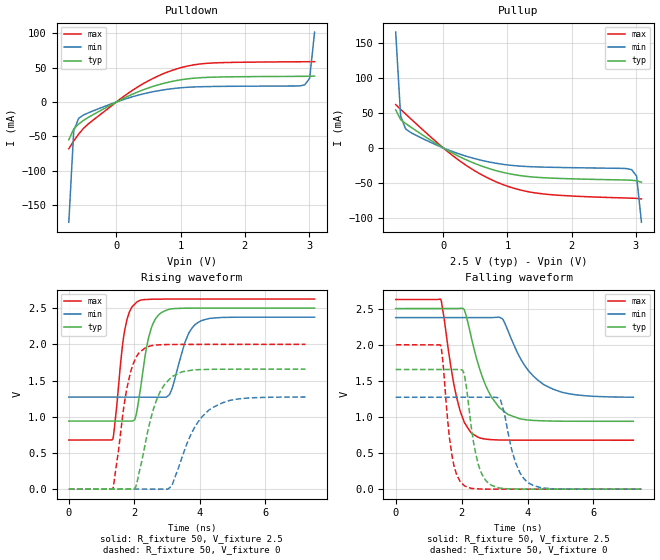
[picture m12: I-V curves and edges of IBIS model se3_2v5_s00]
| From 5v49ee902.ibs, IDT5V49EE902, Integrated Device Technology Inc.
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[Model]   se3_2v5_s00
Model_type   Output
Polarity   Non-Inverting
|   typ   min   max
C_comp   2pF   1.5pF   2.5pF
Vmeas = 1.25V
Rref = 50
Cref = 0
Vref = 1.25V
|   typ   min   max
[Voltage range]   2.5V   2.375V   2.625V
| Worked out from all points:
|   slope of the pulldown table from 0 to 0.375 V, typ, clamps not added: 23.2 ohm
|   slope of the pullup table from 0 to 0.375 V, typ, clamps not added: 21 ohm
|   rising waveform, R_fixture 50, V_fixture 2.5: 20-80 % time 352ps typ, 443ps min, 279ps max; typ from 0.939 V to 2.5 V
|   falling waveform, R_fixture 50, V_fixture 2.5: 20-80 % time 692ps typ, 919ps min, 460ps max; typ from 2.5 V to 0.939 V
|   rising waveform, R_fixture 50, V_fixture 0: 20-80 % time 568ps typ, 793ps min, 399ps max; typ from 0 V to 1.66 V
|   falling waveform, R_fixture 50, V_fixture 0: 20-80 % time 344ps typ, 431ps min, 274ps max; typ from 1.66 V to 0 V
[Pulldown]
|Voltage   I (typ)   I (min)   I (max)
|Note, modeling breaks down at 250mA and above.  This is well beyond the functional   |
|operating range of the device.  Should this scenario occur, catastrophic failure and   |
|possible damage to the device and/or board is of higher concern than the I-V curve   |
|behavior.  The IBIS checker will flag currents in excess of 10A with warnings.  Lines   |
|with currents in excess of 0.35 A have been commented out.  The points still remain|
|available to the user if the user desires to use them.   |
|-2.50000e+00   -4.54709e+01   -3.63694e+01   -6.07959e+01
|-2.42347e+00   -4.32502e+01   -3.46594e+01   -5.77053e+01
|-2.34694e+00   -4.10314e+01   -3.29511e+01   -5.46170e+01
|-2.27041e+00   -3.88148e+01   -3.12446e+01   -5.15313e+01
|-2.19388e+00   -3.66007e+01   -2.95401e+01   -4.84486e+01
|-2.11735e+00   -3.43893e+01   -2.78380e+01   -4.53691e+01
|-2.04082e+00   -3.21809e+01   -2.61384e+01   -4.22934e+01
|-1.96429e+00   -2.99761e+01   -2.44418e+01   -3.92219e+01
|-1.88776e+00   -2.77753e+01   -2.27484e+01   -3.61555e+01
|-1.81122e+00   -2.55791e+01   -2.10589e+01   -3.30948e+01
|-1.73469e+00   -2.33884e+01   -1.93737e+01   -3.00411e+01
|-1.65816e+00   -2.12042e+01   -1.76937e+01   -2.69958e+01
|-1.58163e+00   -1.90279e+01   -1.60198e+01   -2.39607e+01
|-1.50510e+00   -1.68611e+01   -1.43533e+01   -2.09385e+01
|-1.42857e+00   -1.47065e+01   -1.26960e+01   -1.79331e+01
|-1.35204e+00   -1.25675e+01   -1.10500e+01   -1.49501e+01
|-1.27551e+00   -1.04495e+01   -9.41889e+00   -1.19989e+01
|-1.19898e+00   -8.36102e+00   -7.80755e+00   -9.09553e+00
|-1.12245e+00   -6.31683e+00   -6.22400e+00   -6.27207e+00
|-1.04592e+00   -4.34540e+00   -4.68188e+00   -3.60463e+00
|-9.69388e-01   -2.51112e+00   -3.20700e+00   -1.33260e+00
|-8.92857e-01   -9.89892e-01   -1.85502e+00   -2.01598e-01
|-8.16327e-01   -1.92135e-01   -7.61074e-01   -8.24374e-02
-739.8mV  -54.82mA   -174.4mA   -67.73mA
-663.3mV  -39mA      -41.68mA   -56.5mA
-586.7mV  -31.96mA   -23.62mA   -46.47mA
-433.7mV  -22.15mA   -15.6mA    -31.55mA
255.1mV   11.54mA    7.746mA    17.23mA
637.8mV   24.55mA    16.14mA    37.26mA
943.9mV   31.29mA    20.16mA    48.22mA
1.173V    34.28mA    21.72mA    53.44mA
1.48V     36mA       22.52mA    56.56mA
2.934V    37.31mA    24.91mA    58.47mA
3.01V     37.39mA    34.58mA    58.51mA
3.087V    37.69mA    101.5mA    58.57mA
| 3.16327e+00   3.94370e-02   3.90706e-01   5.87161e-02
| 3.23980e+00   5.34568e-02   9.26296e-01   5.92247e-02
| 3.31633e+00   1.87774e-01   1.58657e+00   6.05142e-02
| 3.39286e+00   7.03870e-01   2.30639e+00   6.31621e-02
| 3.46939e+00   1.49288e+00   3.05886e+00   8.17834e-02
| 3.54592e+00   2.39288e+00   3.83148e+00   3.62561e-01
| 3.62245e+00   3.34491e+00   4.61762e+00   1.23059e+00
| 3.69898e+00   4.32602e+00   5.41341e+00   2.35266e+00
| 3.77551e+00   5.32544e+00   6.21640e+00   3.56507e+00
| 3.85204e+00   6.33737e+00   7.02496e+00   4.82041e+00
| 3.92857e+00   7.35834e+00   7.83797e+00   6.10033e+00
| 4.00510e+00   8.38614e+00   8.65458e+00   7.39607e+00
| 4.08163e+00   9.41929e+00   9.47419e+00   8.70278e+00
| 4.15816e+00   1.04567e+01   1.02963e+01   1.00176e+01
| 4.23469e+00   1.14977e+01   1.11206e+01   1.13385e+01
| 4.31122e+00   1.25415e+01   1.19467e+01   1.26642e+01
| 4.38776e+00   1.35879e+01   1.27745e+01   1.39940e+01
| 4.46429e+00   1.46363e+01   1.36036e+01   1.53269e+01
| 4.54082e+00   1.56867e+01   1.44341e+01   1.66626e+01
| 4.61735e+00   1.67386e+01   1.52656e+01   1.80006e+01
| 4.69388e+00   1.77920e+01   1.60982e+01   1.93406e+01
| 4.77041e+00   1.88466e+01   1.69317e+01   2.06823e+01
| 4.84694e+00   1.99024e+01   1.77660e+01   2.20256e+01
| 4.92347e+00   2.09592e+01   1.86011e+01   2.33703e+01
| 5.00000e+00   2.20169e+01   1.94369e+01   2.47161e+01
[Pullup]
|Voltage   I (typ)   I (min)   I (max)
|Note, modeling breaks down at 250mA and above.  This is well beyond the functional   |
|operating range of the device.  Should this scenario occur, catastrophic failure and   |
|possible damage to the device and/or board is of higher concern than the I-V curve   |
|behavior.  The IBIS checker will flag currents in excess of 10A with warnings.  Lines   |
|with currents in excess of 0.35 A have been commented out.  The points still remain|
|available to the user if the user desires to use them.   |
|-2.50000e+00   2.19749e+01   1.80462e+01   2.68494e+01
|-2.42347e+00   2.09176e+01   1.72118e+01   2.55026e+01
|-2.34694e+00   1.98612e+01   1.63782e+01   2.41568e+01
|-2.27041e+00   1.88058e+01   1.55455e+01   2.28121e+01
|-2.19388e+00   1.77516e+01   1.47137e+01   2.14686e+01
|-2.11735e+00   1.66986e+01   1.38831e+01   2.01266e+01
|-2.04082e+00   1.56470e+01   1.30536e+01   1.87861e+01
|-1.96429e+00   1.45970e+01   1.22255e+01   1.74474e+01
|-1.88776e+00   1.35488e+01   1.13989e+01   1.61108e+01
|-1.81122e+00   1.25028e+01   1.05741e+01   1.47767e+01
|-1.73469e+00   1.14592e+01   9.75133e+00   1.34454e+01
|-1.65816e+00   1.04186e+01   8.93094e+00   1.21176e+01
|-1.58163e+00   9.38151e+00   8.11336e+00   1.07941e+01
|-1.50510e+00   8.34872e+00   7.29916e+00   9.47586e+00
|-1.42857e+00   7.32129e+00   6.48907e+00   8.16447e+00
|-1.35204e+00   6.30078e+00   5.68413e+00   6.86214e+00
|-1.27551e+00   5.28938e+00   4.88577e+00   5.57245e+00
|-1.19898e+00   4.29063e+00   4.09609e+00   4.30150e+00
|-1.12245e+00   3.31046e+00   3.31840e+00   3.06092e+00
|-1.04592e+00   2.35988e+00   2.55815e+00   1.87698e+00
|-9.69388e-01   1.46255e+00   1.82528e+00   8.26188e-01
|-8.92857e-01   6.79691e-01   1.14020e+00   1.77018e-01
|-8.16327e-01   1.78301e-01   5.50929e-01   7.20286e-02
-739.8mV  54.64mA    166.3mA    62.19mA
-663.3mV  40.61mA    45.96mA    55.4mA
-586.7mV  35.13mA    27.42mA    48.78mA
-204.1mV  11.53mA    8.292mA    16.47mA
255.1mV   -12.67mA   -8.857mA   -18.54mA
561.2mV   -24.84mA   -17.08mA   -36.7mA
943.9mV   -35.45mA   -23.78mA   -53.18mA
1.25V     -40.42mA   -26.48mA   -61.53mA
1.556V    -42.81mA   -27.59mA   -66.09mA
2.934V    -46.44mA   -31.28mA   -72.19mA
3.01V     -47.21mA   -40.39mA   -72.48mA
3.087V    -49.28mA   -106.7mA   -73.28mA
| 3.16327e+00   -5.35776e-02   -4.94236e-01   -7.58575e-02
| 3.23980e+00   -6.85824e-02   -1.43626e+00   -8.09810e-02
| 3.31633e+00   -2.12479e-01   -2.71822e+00   -8.81300e-02
| 3.39286e+00   -1.02359e+00   -4.15794e+00   -9.69441e-02
| 3.46939e+00   -2.55073e+00   -5.67974e+00   -1.18777e-01
| 3.54592e+00   -4.38708e+00   -7.25021e+00   -4.69271e-01
| 3.62245e+00   -6.35927e+00   -8.85247e+00   -2.14689e+00
| 3.69898e+00   -8.40369e+00   -1.04769e+01   -4.62063e+00
| 3.77551e+00   -1.04921e+01   -1.21177e+01   -7.36117e+00
| 3.85204e+00   -1.26099e+01   -1.37710e+01   -1.02197e+01
| 3.92857e+00   -1.47486e+01   -1.54342e+01   -1.31429e+01
| 4.00510e+00   -1.69029e+01   -1.71053e+01   -1.61066e+01
| 4.08163e+00   -1.90692e+01   -1.87829e+01   -1.90980e+01
| 4.15816e+00   -2.12452e+01   -2.04660e+01   -2.21093e+01
| 4.23469e+00   -2.34289e+01   -2.21537e+01   -2.51357e+01
| 4.31122e+00   -2.56192e+01   -2.38455e+01   -2.81738e+01
| 4.38776e+00   -2.78148e+01   -2.55407e+01   -3.12215e+01
| 4.46429e+00   -3.00151e+01   -2.72389e+01   -3.42769e+01
| 4.54082e+00   -3.22195e+01   -2.89399e+01   -3.73388e+01
| 4.61735e+00   -3.44273e+01   -3.06432e+01   -4.04061e+01
| 4.69388e+00   -3.66382e+01   -3.23486e+01   -4.34782e+01
| 4.77041e+00   -3.88519e+01   -3.40560e+01   -4.65543e+01
| 4.84694e+00   -4.10679e+01   -3.57652e+01   -4.96340e+01
| 4.92347e+00   -4.32862e+01   -3.74759e+01   -5.27168e+01
| 5.00000e+00   -4.55064e+01   -3.91880e+01   -5.58024e+01
[Ramp]
|   typ   min   max
dV/dt_r   0.936/0.352n   0.663/0.443n   1.168/0.279n
dV/dt_f   0.939/0.692n   0.665/0.919n   1.172/0.46n
R_load =   50
[Rising Waveform]
R_fixture = 50
V_fixture = 2.5   |Vcc_typ
V_fixture_min = 2.375 |Vcc_min
V_fixture_max = 2.625 |Vcc_max
C_fixture = 0.0p
| Time   typ   min   max
0s        939.3mV    1.271V     677.7mV
1.339ns   939.3mV    1.271V     689.1mV
1.7ns     939.3mV    1.271V     2.184V
2.089ns   1.104V     1.271V     2.589V
2.429ns   2.082V     1.271V     2.621V
2.816ns   2.435V     1.27V      2.625V
3.073ns   2.485V     1.306V     2.625V
3.534ns   2.499V     2.017V     2.625V
3.97ns    2.5V       2.309V     2.625V
7.5ns     2.5V       2.375V     2.625V
[Falling Waveform]
R_fixture = 50
V_fixture = 2.5   |Vcc_typ
V_fixture_min = 2.375 |Vcc_min
V_fixture_max = 2.625 |Vcc_max
C_fixture = 0.0p
| Time   typ   min   max
0s        2.5V       2.375V     2.625V
1.37ns    2.5V       2.375V     2.627V
1.951ns   2.502V     2.375V     1.087V
2.082ns   2.484V     2.375V     924.2mV
2.457ns   1.802V     2.375V     729.3mV
2.902ns   1.279V     2.375V     685.4mV
3.411ns   1.033V     2.19V      678.8mV
3.913ns   963.2mV    1.713V     678mV
4.495ns   945.1mV    1.446V     677.9mV
7.213ns   939.5mV    1.273V     677.8mV
[Rising Waveform]
R_fixture = 50
V_fixture = 0
C_fixture = 0.0p
| Time   typ   min   max
0s        1.586nV    7.942nV    136.5pV
1.35ns    -13.68nV   8.225nV    10.74mV
1.87ns    -174.4uV   30.88nV    1.592V
2.044ns   31.78mV    -4.071nV   1.815V
2.37ns    712.7mV    -751.4nV   1.961V
2.798ns   1.354V     52.37uV    1.994V
3.453ns   1.62V      436.7mV    1.999V
3.971ns   1.65V      944.1mV    1.999V
4.67ns    1.656V     1.188V     1.999V
7.222ns   1.657V     1.272V     1.999V
[Falling Waveform]
R_fixture = 50
V_fixture = 0
C_fixture = 0.0p
| Time   typ   min   max
0s        1.657V     1.272V     1.999V
1.361ns   1.657V     1.272V     1.993V
1.704ns   1.657V     1.272V     479.9mV
2.095ns   1.557V     1.272V     43.22mV
2.5ns     353.6mV    1.272V     3.424mV
2.914ns   51.58mV    1.273V     518.1uV
3.183ns   13.96mV    1.23V      269.2uV
3.638ns   1.877mV    365.6mV    182.8uV
4.027ns   517.8uV    88.67mV    148.4uV
7.458ns   108.2uV    233.5uV    54.01uV
